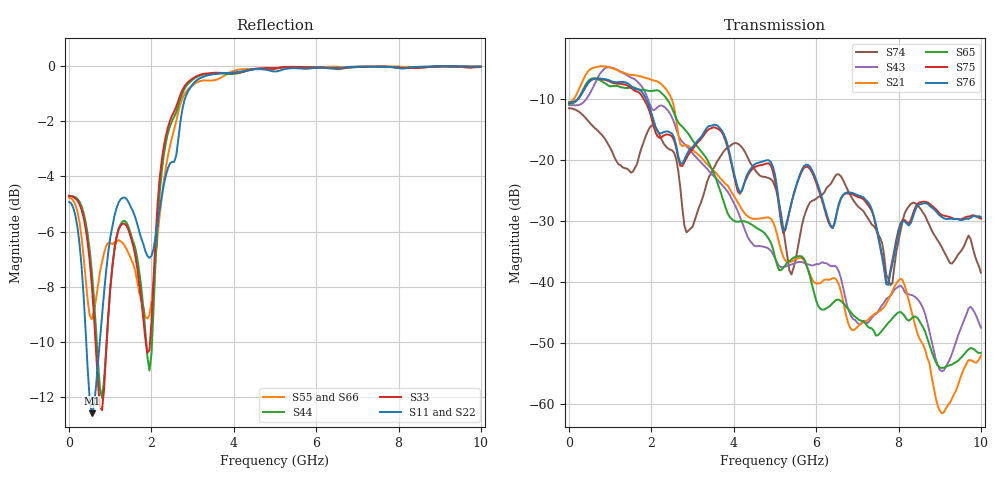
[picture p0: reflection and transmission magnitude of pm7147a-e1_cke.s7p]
# GHz S DB R 50
! S-Parameters data
! Freq  dbS11  angS11  dbS12  angS12  dbS13  angS13  dbS14  angS14
!  dbS15  angS15  dbS16  angS16  dbS17  angS17  dbS21  angS21
!  dbS22  angS22  dbS23  angS23  dbS24  angS24  dbS25  angS25
!  dbS26  angS26  dbS27  angS27  dbS31  angS31  dbS32  angS32
!  dbS33  angS33  dbS34  angS34  dbS35  angS35  dbS36  angS36
!  dbS37  angS37  dbS41  angS41  dbS42  angS42  dbS43  angS43
!  dbS44  angS44  dbS45  angS45  dbS46  angS46  dbS47  angS47
!  dbS51  angS51  dbS52  angS52  dbS53  angS53  dbS54  angS54
!  dbS55  angS55  dbS56  angS56  dbS57  angS57  dbS61  angS61
!  dbS62  angS62  dbS63  angS63  dbS64  angS64  dbS65  angS65
!  dbS66  angS66  dbS67  angS67  dbS71  angS71  dbS72  angS72
!  dbS73  angS73  dbS74  angS74  dbS75  angS75  dbS76  angS76
!  dbS77  angS77
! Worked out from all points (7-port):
!   279 points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, 1 Hz to 10 GHz, reference 50 ohm
!   strongest paths, dB at 1 Hz, 7.943 MHz, 3.05 GHz, 6.55 GHz, 10 GHz:
!     S76: -10.6, -10.6, -17.5, -27.4, -29.3
!     S75: -10.6, -10.6, -17.8, -27.2, -29.6
!     S65: -10.8, -10.8, -17.3, -42.9, -51.6
!     S21: -10.5, -10.5, -18.7, -40.4, -52.1
!     S43: -11.0, -11.0, -19.3, -38.3, -47.5
!     S74: -11.5, -11.5, -29.9, -22.4, -38.5
!   lowest |S11| = -12.6 dB at 550 MHz (marker M1), VSWR 1.61, Z = 31 + j0.695 ohm
!   |S11| at or under -10 dB: 415.7 MHz to 743.9 MHz (328.2 MHz wide, 56.6 % of centre)
